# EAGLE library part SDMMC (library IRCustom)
SD MMC Card holder 4UCON part #06132 - easy to solder
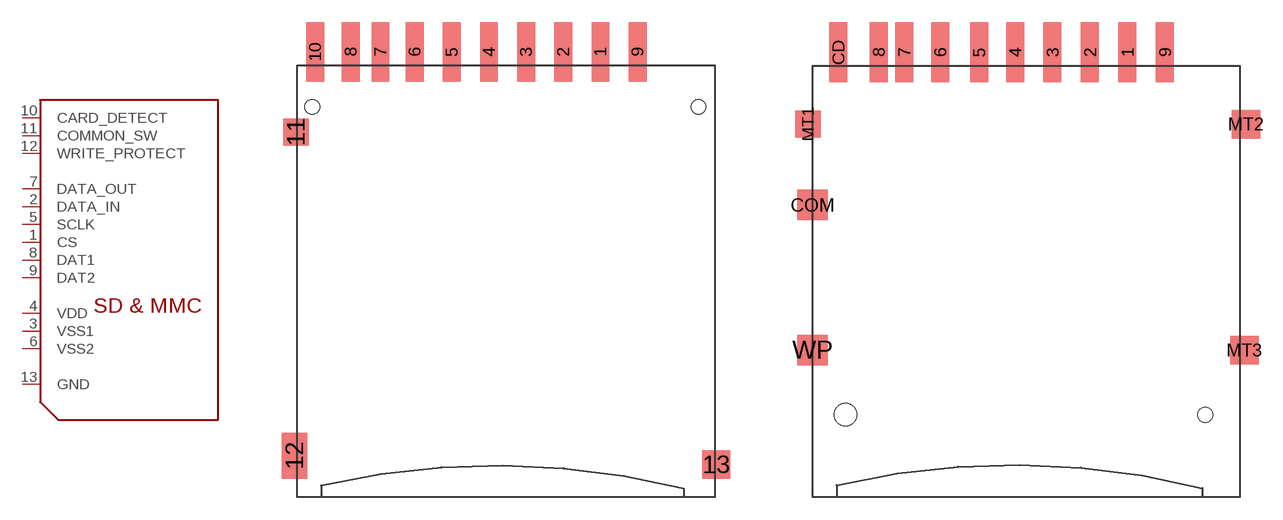
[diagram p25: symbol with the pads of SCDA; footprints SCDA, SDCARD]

Designator prefix -

## SDMMCSCDA  [SCDA]
1  CS  in
2  DATA_IN  in
3  VSS1  sup
4  VDD  sup
5  SCLK  in
6  VSS2  sup
7  DATA_OUT  out
8  DAT1
9  DAT2
10  CARD_DETECT  pas
11  COMMON_SW  pas
12  WRITE_PROTECT  pas
13  GND  sup

## SDMMC18650  [SDCARD]
1  CS  in
2  DATA_IN  in
3  VSS1  sup
4  VDD  sup
5  SCLK  in
6  VSS2  sup
7  DATA_OUT  out
8  DAT1
9  DAT2
CD  CARD_DETECT  pas
COM  COMMON_SW  pas
MT1  GND  sup
WP  WRITE_PROTECT  pas

## SDMMC06132  [06132]
1  CS  in
2  DATA_IN  in
3  VSS1  sup
4  VDD  sup
5  SCLK  in
6  VSS2  sup
7  DATA_OUT  out
8  DAT1
9  DAT2
CD  CARD_DETECT  pas
GP  GND  sup
GP3  COMMON_SW  pas
WP  WRITE_PROTECT  pas

## Footprint SCDA (pad centres in mm)
smd 1.2 x 4: 1 6.4,3.7; 2 3.9,3.7; 3 1.4,3.7; 4 -1.1,3.7; 5 -3.6,3.7; 6 -6.1,3.7; 7 -8.4,3.7; 8 -10.4,3.7; 9 8.9,3.7; 10 -12.8,3.7
smd 1.7 x 1.8: 11 -14.1,-1.7
smd 1.7 x 3.1: 12 -14.2,-23.5
smd 1.9 x 1.9: 13 14.2,-24.1
hole 1 at -13,0
hole 1 at 13,0

## Footprint SDCARD (pad centres in mm)
smd 1.2 x 4: 1 6.8,0.89; 2 4.3,0.89; 3 1.8,0.89; 4 -0.7,0.89; 5 -3.1,0.89; 6 -5.7,0.89; 7 -8.1,0.89; 8 -9.8,0.89; 9 9.3,0.89; CD -12.5,0.89
smd 2.032 x 2.032: COM -14.2,-9.3; WP -14.2,-19
smd 1.7 x 1.8: MT1 -14.5,-3.91
smd 1.9 x 1.9: MT2 14.7,-3.91; MT3 14.6,-19.01
hole 1.5 at -12,-23.31
hole 1 at 12,-23.31

## Footprint 06132 (pad centres in mm)
smd 1.2 x 4: 1 6.9,0.9; 2 4.4,0.9; 3 1.9,0.9; 4 -0.6,0.9; 5 -3.1,0.9; 6 -5.6,0.9; 7 -8.1,0.9; 9 9.4,0.9
smd 0.7 x 4: 8 -9.7,0.9; CD -11,0.9; WP -12.2,0.9
smd 2 x 2.8: GP -13.8,-21.8; GP2 14.1,-21.8; GP3 11.7,-0.9; GP4 -13.9,-1
hole 1.1 at -11.6,-2.1
hole 1.6 at 9.5,-2.1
